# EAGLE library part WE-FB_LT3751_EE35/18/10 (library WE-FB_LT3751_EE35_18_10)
Flyback Converter WE-FB for LT3751 - designd for LT3751
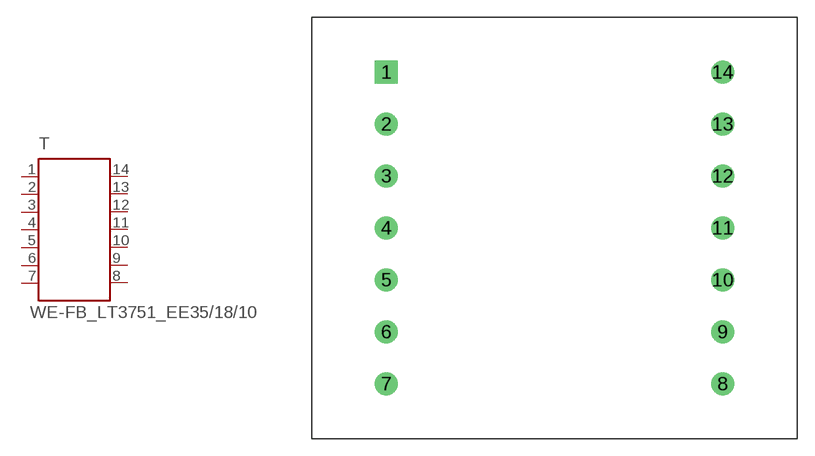
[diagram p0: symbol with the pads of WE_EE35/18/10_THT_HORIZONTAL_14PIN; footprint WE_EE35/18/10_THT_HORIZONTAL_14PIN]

Designator prefix T

## WE-FB_LT3751_EE35/18/10-750310349 (MPN: 750310349; OC_FARNELL: 1748694; OC_NEWARK: 34R6107; PACKAGE: EE35_18_10; SUPPLIER: Würth Elektronik eiSos GmbH), WE-FB_LT3751_EE35/18/10-750310355 (MPN: 750310355; OC_FARNELL: 1748696; OC_NEWARK: 34R6108; PACKAGE: EE35_18_10; SUPPLIER: Würth Elektronik eiSos GmbH)  [WE_EE35/18/10_THT_HORIZONTAL_14PIN]
1  1  pas
2  2  pas
3  3  pas
4  4  pas
5  5  pas
6  6  pas
7  7  pas
8  8  pas
9  9  pas
10  10  pas
11  11  pas
12  12  pas
13  13  pas
14  14  pas

## Footprint WE_EE35/18/10_THT_HORIZONTAL_14PIN (pad centres in mm)
Transformer, EE35/18/10 THT Horizontal 14Pin
drill 1.32 square: 1 -14.55,13.5
drill 1.32: 2 -14.55,9; 3 -14.55,4.5; 4 -14.55,0; 5 -14.55,-4.5; 6 -14.55,-9; 7 -14.55,-13.5; 8 14.55,-13.5; 9 14.55,-9; 10 14.55,-4.5; 11 14.55,0; 12 14.55,4.5; 13 14.55,9; 14 14.55,13.5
